TYPE ST_EL5131_Setting :
STRUCT
	SetDigitalOutput				:	BIT;
//	EnableThresholdsOutput			:	BIT;
	SetTristate						:	BIT;
	DisableThresholdsCw				:	BIT;
	DisableThresholdsCcw			:	BIT;
END_STRUCT
END_TYPE
